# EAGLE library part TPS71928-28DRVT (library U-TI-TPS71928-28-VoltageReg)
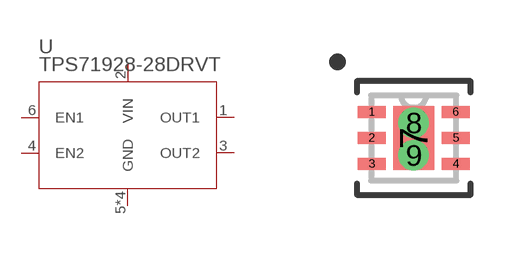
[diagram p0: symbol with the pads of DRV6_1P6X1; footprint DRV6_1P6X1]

Designator prefix U

## TPS71928-28DRVT (MANUFACTURER_PART_NUMBER: TPS7192828DRVT; VENDOR: Texas Instruments)  [DRV6_1P6X1]
1  OUT1  pwr
2  VIN  pwr
3  OUT2  pwr
4  EN2  pas
5  GND  pwr
6  EN1  pas
7  GND  pwr
8  GND  pwr
9  GND  pwr

## Footprint DRV6_1P6X1 (pad centres in mm)
smd 0.7 x 0.3: 1 -1.05,0.65; 2 -1.05,0; 3 -1.05,-0.65; 4 1.05,-0.65; 5 1.05,0; 6 1.05,0.65
smd 1.016 x 1.6: 7 0,0
drill 0.254 pad 0.508: 8 0,0.375; 9 0,-0.438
